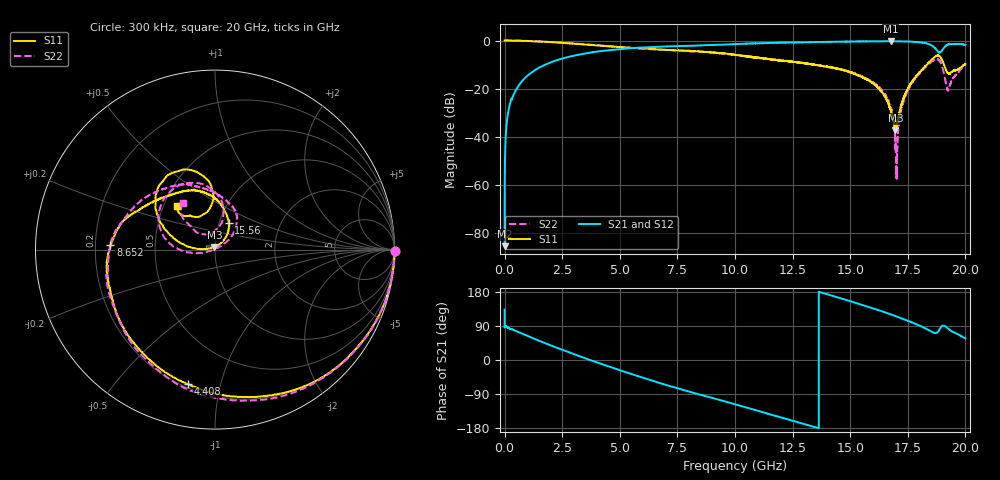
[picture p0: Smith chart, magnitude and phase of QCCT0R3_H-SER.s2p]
!{QCCT0R3}
!Johanson Technology Inc.
!www.johansontechnology.com
!Test Board Conditions:
!Substrate Type  RO4350B
!Substrate Thickness  20 mil
!Substrate Dk  3.66
!TL Type: GCPW
!TL Trace Width  34 mil
!TL Gap  10 mil
!Electrode orientation  Horizontal
!DUT TOPOLOGY	SERIES
!Mounting Pad LxW  26x52 mil
# MHz S  dB  R 50
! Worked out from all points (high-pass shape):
!   20001 points, 300 kHz to 20 GHz, reference 50 ohm
!   highest |S21| = -0.26 dB at 16.76 GHz (marker M1); lowest = -85.7 dB at 300 kHz (marker M2)
!   |S21| within 3 dB of the highest: 5.408 GHz to 18.69 GHz (13.28 GHz wide, 110 % of centre); 19.05 GHz to end of sweep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
!   lowest |S11| = -37.4 dB at 16.96 GHz (marker M3), VSWR 1.03, Z = 49.6 + j1.29 ohm
!   |S11| at or under -10 dB: 13.40006 GHz to 13.40018 GHz (114 kHz wide, 0.00085 % of centre); 13.41 GHz to 18.34 GHz (4.928 GHz wide, 31 % of centre); 19.07 GHz to 19.96 GHz (895.2 MHz wide, 4.59 % of centre)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
!   |S22| runs from -57.6 to 0.0 dB; largest |S21 - S12| = 0.014
!   S11 on the Smith chart (normalised r, x): 300 kHz: open; 4.408 GHz: 0.22, -0.80; 8.652 GHz: 0.26, +0.02; 15.56 GHz: 1.11, +0.34; 20 GHz: 0.59, +0.32
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0.3  0.02 -0.3  -85.69 133.0  -81.20 77.8  0.01 -0.4
102.298  -0.00 -2.9  -33.44 86.8  -33.41 86.6  0.00 -3.0
139.298  -0.01 -3.9  -30.78 85.7  -30.73 85.9  -0.01 -3.9
520.292  -0.04 -13.7  -20.13 75.9  -20.11 76.0  -0.05 -13.7
1516.277  -0.41 -39.0  -11.22 50.4  -11.20 50.4  -0.40 -39.5
3334.25  -1.55 -79.2  -5.69 8.2  -5.67 8.2  -1.48 -83.9
4408.234  -2.32 -101.3  -4.16 -14.6  -4.15 -14.7  -2.27 -107.8
6667.2  -3.69 -146.5  -2.62 -59.5  -2.60 -59.3  -3.79 -151.8
8652.17  -4.68 177.5  -1.98 -94.3  -1.97 -94.2  -4.74 175.0
10000.15  -5.93 157.0  -1.50 -116.8  -1.46 -116.9  -5.95 150.4
13334.1  -9.92 99.3  -0.66 -174.8  -0.70 -174.8  -9.90 91.6
15560.07  -15.45 63.1  -0.35 144.8  -0.39 144.7  -15.24 48.4
16667.05  -26.48 48.3  -0.28 122.2  -0.33 122.5  -25.13 32.6
16757.05  -28.93 51.7  -0.26 120.5  -0.30 120.5  -27.93 30.8
16962.05  -37.38 105.9  -0.31 116.0  -0.30 116.1  -42.23 54.6
17057.04  -33.37 151.4  -0.31 113.8  -0.30 114.1  -41.87 177.6
17184.04  -28.01 172.1  -0.33 110.9  -0.35 111.2  -30.42 -165.6
17391.04  -22.16 177.9  -0.39 106.3  -0.39 106.3  -23.12 -165.2
18085.03  -12.48 164.9  -0.85 88.7  -0.81 88.4  -12.87 176.3
18814.02  -6.21 118.8  -4.59 74.7  -4.56 74.7  -7.85 114.8
19261.01  -13.70 108.9  -1.61 82.3  -1.59 82.6  -20.60 115.4
20000  -9.83 130.9  -1.85 57.4  -1.93 57.1  -9.99 124.2
